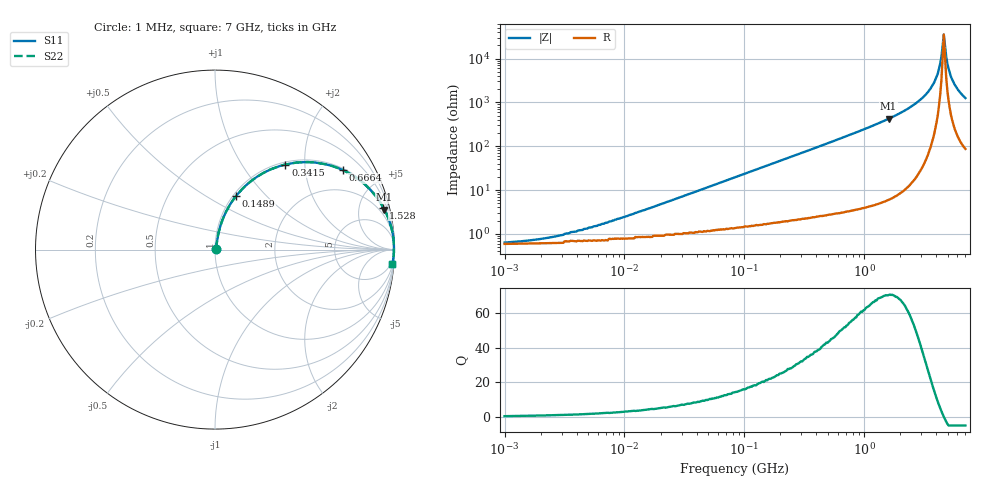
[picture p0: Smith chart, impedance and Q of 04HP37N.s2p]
# MHz S MA R 50
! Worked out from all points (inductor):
!   385 points, 1 MHz to 7 GHz, reference 50 ohm
!   read as one part in series: L = 37 nH near 10.27 MHz
!   highest Q = 70.7 at 1.6 GHz (marker M1), where L = 42.1 nH
!   self-resonance near 4.622 GHz
!   S11 on the Smith chart (normalised r, x): 1 MHz: 1.01, +0.00; 148.9 MHz: 1.03, +0.69; 341.5 MHz: 1.05, +1.60; 666.4 MHz: 1.06, +3.16; 1.528 GHz: 1.11, +7.98; 7 GHz: 3, -25
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1  0.006185 21.8  0.994 -0.1  0.994 -0.1  0.006185 21.8
4.374  0.012 55.5  0.993 -0.6  0.993 -0.6  0.012 55.5
19.575  0.046 76.1  0.99 -2.6  0.99 -2.6  0.046 76.1
85.617  0.193 74.9  0.968 -11.1  0.968 -11.1  0.193 74.9
148.895  0.323 68.4  0.931 -18.8  0.931 -18.8  0.323 68.4
341.475  0.615 50.4  0.771 -38.0  0.771 -38.0  0.615 50.4
365.931  0.642 48.5  0.749 -39.9  0.749 -39.9  0.642 48.5
666.414  0.838 32.0  0.53 -56.9  0.53 -56.9  0.838 32.0
1528.346  0.967 14.0  0.242 -75.2  0.242 -75.2  0.967 14.0
1600.473  0.97 13.3  0.229 -75.9  0.229 -75.9  0.97 13.3
1637.803  0.972 12.9  0.223 -76.3  0.223 -76.3  0.972 12.9
2657.911  0.992 6.2  0.108 -82.7  0.108 -82.7  0.992 6.2
3586.848  0.997 2.7  0.048 -84.6  0.048 -84.6  0.997 2.7
3843.73  0.997 2.0  0.035 -84.2  0.035 -84.2  0.997 2.0
4215.081  0.997 1.0  0.017 -80.7  0.017 -80.7  0.997 1.0
4414.002  0.997 0.5  0.009116 -72.6  0.009116 -72.6  0.997 0.5
4622.31  0.997 0.0  0.002813 -3.5  0.002813 -3.5  0.997 0.0
4840.449  0.997 -0.5  0.008889 69.9  0.008889 69.9  0.997 -0.5
4953.349  0.997 -0.7  0.013 75.6  0.013 75.6  0.997 -0.7
5308.095  0.996 -1.5  0.026 80.9  0.026 80.9  0.996 -1.5
6095.627  0.994 -3.0  0.052 82.3  0.052 82.3  0.994 -3.0
7000  0.991 -4.5  0.079 81.5  0.079 81.5  0.991 -4.5
